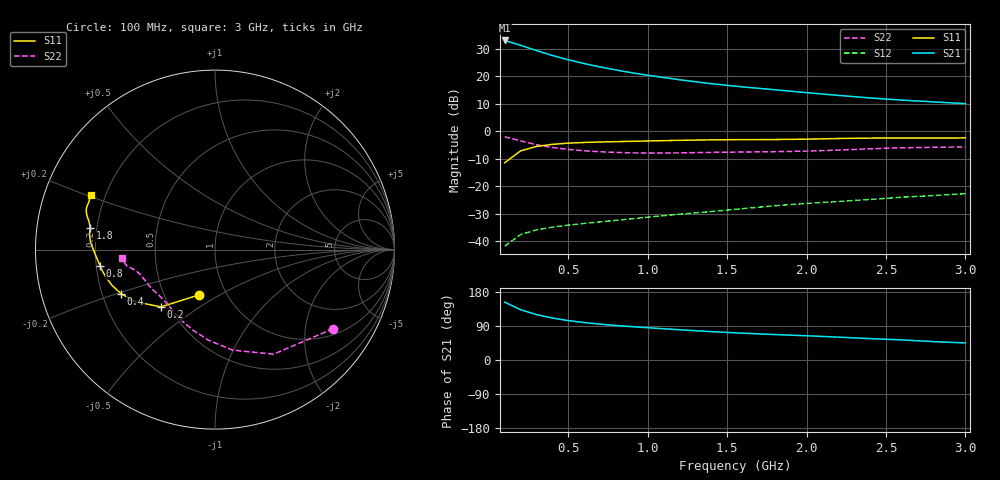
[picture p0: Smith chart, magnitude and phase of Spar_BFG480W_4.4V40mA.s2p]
! Filename: 4_440BFG480.001
! Title: BFG480W
! Bias: Vce=4.4V; Ic=40mA
! Company: NXP Semiconductors NL
! User: Quality&Reliability T&D
! Measure time: 10 Nov 1999 / 12:05:49
#  MHz  S  MA  R 50
! Freq  S11  S21  S12  S22  :
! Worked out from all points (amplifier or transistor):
!   20 points, 100 MHz to 3 GHz, reference 50 ohm
!   highest |S21| = 33.0 dB at 100 MHz (marker M1)
!   |S21| within 3 dB of that: start of sweep to 265 MHz
!   unconditionally stable (mu >= 1): 1.039 GHz to end of sweep
!   at 400 MHz: K = 0.60, MSG = 31.2 dB, |S12| = -34.9 dB
!   at 1.2 GHz: K = 1.04, MAG = 23.2 dB, |S12| = -30.2 dB
!   at 3 GHz: K = 1.06, MAG = 14.8 dB, |S12| = -22.7 dB
!   S11 on the Smith chart (normalised r, x): 100 MHz: 0.75, -0.40; 200 MHz: 0.45, -0.36; 400 MHz: 0.28, -0.21; 800 MHz: 0.22, -0.07; 1.8 GHz: 0.17, +0.08; 3 GHz: 0.14, +0.20
100  0.266 -109.0  44.71 152.6  0.008127 62.0  0.7923 -33.8
200  0.4384 -133.3  36.56 132.9  0.01321 54.3  0.6679 -60.7
300  0.5289 -146.6  29.29 119.8  0.01609 50.2  0.5688 -80.0
400  0.5774 -154.7  23.84 110.7  0.018 49.0  0.506 -94.2
500  0.6068 -160.7  19.94 104.1  0.0196 49.5  0.4668 -104.9
600  0.6245 -165.2  16.99 98.8  0.02105 50.9  0.4413 -113.2
700  0.6367 -168.8  14.76 94.6  0.02246 52.9  0.4238 -119.8
800  0.6464 -171.9  13 91.0  0.02397 54.9  0.412 -125.4
900  0.6555 -174.6  11.57 88.0  0.02555 57.2  0.4046 -130.2
1000  0.6649 -177.0  10.42 85.2  0.02738 59.0  0.4012 -134.5
1200  0.6829 179.0  8.628 79.9  0.03096 62.3  0.4039 -141.8
1400  0.6967 176.0  7.321 74.8  0.03463 64.9  0.4124 -147.3
1600  0.7042 173.2  6.386 70.7  0.03916 67.2  0.4186 -151.4
1800  0.706 170.3  5.675 67.2  0.0442 69.0  0.4251 -155.6
2000  0.7171 167.7  5.024 64.0  0.04859 70.7  0.4349 -160.4
2200  0.7373 165.2  4.485 60.3  0.05269 71.5  0.454 -164.8
2400  0.7503 163.2  4.024 56.4  0.05733 71.7  0.4793 -167.7
2600  0.7533 161.5  3.678 53.0  0.06314 71.7  0.4996 -169.6
2800  0.7512 159.1  3.415 48.5  0.06781 70.9  0.5098 -171.7
3000  0.7564 156.4  3.169 45.0  0.07306 70.6  0.5177 -174.8
